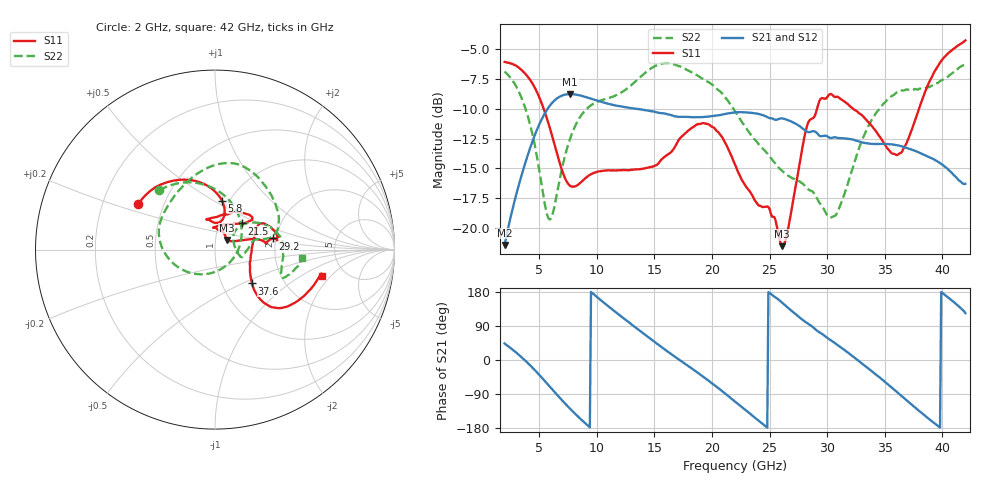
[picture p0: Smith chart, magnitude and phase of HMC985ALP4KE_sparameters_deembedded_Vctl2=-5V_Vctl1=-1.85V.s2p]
!s2p File: Measurements: S11, S21, S12, S22
# GHz S dB R 50.0
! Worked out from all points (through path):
!   401 points, 2 GHz to 42 GHz, reference 50 ohm
!   highest |S21| = -8.77 dB at 7.7 GHz (marker M1); lowest = -21.4 dB at 2 GHz (marker M2)
!   lowest |S11| = -21.5 dB at 26.1 GHz (marker M3), VSWR 1.18, Z = 56.6 + j6.06 ohm
!   |S11| at or under -10 dB: 5.392 GHz to 29.12 GHz (23.73 GHz wide, 138 % of centre); 32.26 GHz to 37.97 GHz (5.714 GHz wide, 16.3 % of centre)
!   |S22| runs from -19.3 to -6.2 dB; largest |S21 - S12| = 0.00037
!   S11 on the Smith chart (normalised r, x): 2 GHz: 0.36, +0.24; 5.8 GHz: 0.93, +0.55; 21.5 GHz: 1.29, +0.39; 29.2 GHz: 1.92, +0.27; 37.6 GHz: 1.39, -0.57; 42 GHz: 3.37, -1.57
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2  -6.06 149.2  -21.43 43.5  -21.44 43.5  -6.87 133.3
3.2  -6.51 130.1  -16.52 14.6  -16.52 14.6  -8.49 102.5
4.4  -7.84 107.9  -12.79 -19.7  -12.79 -19.7  -12.06 61.7
5.8  -11.20 81.9  -9.90 -66.0  -9.91 -66.0  -19.19 -35.4
7.7  -16.48 84.1  -8.77 -129.2  -8.77 -129.2  -12.47 -158.9
8.7  -16.11 96.3  -8.91 -158.6  -8.92 -158.6  -10.48 176.2
10.2  -15.26 103.1  -9.36 161.7  -9.36 161.7  -9.35 154.0
12.2  -15.16 105.9  -9.82 113.1  -9.83 113.1  -8.59 128.5
15.4  -14.53 83.6  -10.34 39.1  -10.35 39.1  -6.28 83.0
18.3  -11.58 49.1  -10.71 -23.4  -10.71 -23.4  -6.97 50.0
21.5  -13.57 44.2  -10.37 -97.3  -10.38 -97.3  -9.48 13.6
22  -14.68 51.0  -10.31 -109.8  -10.31 -109.8  -10.20 12.1
24.1  -18.14 91.8  -10.44 -161.4  -10.45 -161.3  -13.03 13.3
26.1  -21.54 39.5  -10.81 150.9  -10.82 150.9  -15.22 -3.4
28.7  -10.81 6.5  -11.89 88.4  -11.90 88.4  -16.92 -13.6
29.2  -9.72 11.0  -12.13 75.4  -12.14 75.5  -17.69 -10.0
30.8  -8.99 14.6  -12.42 41.6  -12.42 41.6  -18.86 27.1
33  -10.52 29.4  -12.82 -8.5  -12.82 -8.5  -12.70 39.5
35.4  -13.51 7.4  -12.97 -67.5  -12.97 -67.4  -9.11 17.4
37.6  -11.07 -42.4  -13.52 -124.5  -13.53 -124.5  -8.34 -5.8
39.8  -6.12 -41.1  -14.56 -178.3  -14.56 -178.2  -7.68 -22.3
42  -4.26 -13.7  -16.30 123.7  -16.31 123.7  -6.21 -5.2
